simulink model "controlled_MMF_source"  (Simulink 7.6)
settings: Solver=ode15s  StartTime=0.0  StopTime=50  RelTol=1e-3
StopFcn:
  | load MMF_variable_pos_vit.mat
  | close all
  | plotyy(x(1,:),x(2,:),x(1,:),x(3,:))
  | grid
  | title('Position et vitesse de la masse')
  | 
  | figure
  | load MMF_variable_flux_MMF.mat
  | plotyy(y(1,:),y(2,:),y(1,:),y(3,:))
  | grid
  | title('Flux magnétique et MMF')
  | delete *.mat
undefined symbols (not defined in the file or in its folder): sigbuilder_block
libraries: fl_lib x12, nesl_utility x6

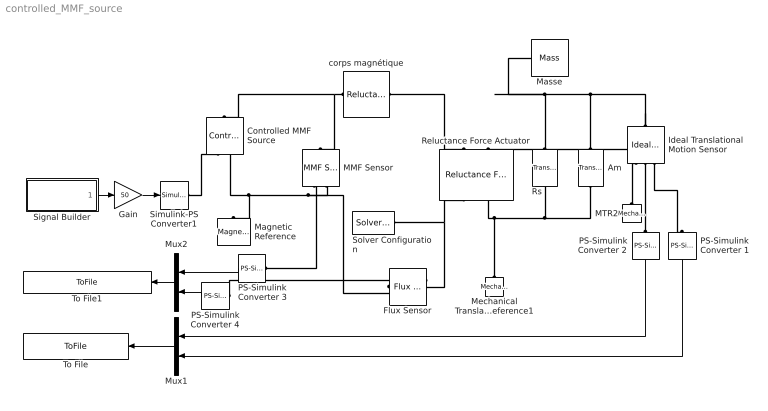
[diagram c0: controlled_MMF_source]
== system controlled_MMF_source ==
  Am : fl_lib/Mechanical/Translational Elements/Translational Damper  DialogController=NetworkEngine.DynNeDlgSource  SystemSampleTime=-1  D=10 N/(m/s)  f_Log=off  v_Log=off  LocalVarNames=|force|rel_velocity|power  LocalVarDescs=|Damping force (N)|Damper relative velocity (m/s)|Power dissipated in the damper (W)  LocalVarLogging=[0 0 0]
  Controlled MMF Source : fl_lib/Magnetic/Magnetic Sources/Controlled MMF Source  DialogController=NetworkEngine.DynNeDlgSource  SystemSampleTime=-1  phi_Log=off  mmf_Log=off  LocalVarNames=|phi|mmf  LocalVarDescs=|phi|mmf  LocalVarLogging=[0 0]
  Flux Sensor : fl_lib/Magnetic/Magnetic Sensors/Flux Sensor  DialogController=NetworkEngine.DynNeDlgSource  SystemSampleTime=-1  phi_Log=off  mmf_Log=off  LocalVarNames=|phi|mmf  LocalVarDescs=|phi|mmf  LocalVarLogging=[0 0]
  Gain : Gain  Gain=50
  Ideal Translational Motion Sensor : fl_lib/Mechanical/Mechanical Sensors/Ideal Translational Motion Sensor  DialogController=NetworkEngine.DynNeDlgSource  SystemSampleTime=-1  offset=5 mm  v_Log=off  f_Log=off  x_Log=off  LocalVarNames=|v|f|x  LocalVarDescs=|v|f|x  LocalVarLogging=[]
  MMF Sensor : fl_lib/Magnetic/Magnetic Sensors/MMF Sensor  DialogController=NetworkEngine.DynNeDlgSource  SystemSampleTime=-1  phi_Log=off  mmf_Log=off  LocalVarNames=|phi|mmf  LocalVarDescs=|phi|mmf  LocalVarLogging=[0 0]
  MTR2 : fl_lib/Mechanical/Translational Elements/Mechanical Translational Reference  Tag=Factory Generic  DialogController=NetworkEngine.DynNeDlgSource  SystemSampleTime=-1  f_Log=off  LocalVarNames=|f  LocalVarDescs=|f  LocalVarLogging=[]
  Magnetic Reference : fl_lib/Magnetic/Magnetic Elements/Magnetic Reference  DialogController=NetworkEngine.DynNeDlgSource  SystemSampleTime=-1  phi_Log=off  LocalVarNames=|phi  LocalVarDescs=|phi  LocalVarLogging=0
  Masse : fl_lib/Mechanical/Translational Elements/Mass  DialogController=NetworkEngine.DynNeDlgSource  SystemSampleTime=-1  mass=1 kg  initial_velocity=0 m/s  f_Log=off  LocalVarNames=|force|velocity  LocalVarDescs=|Inertia force (N)|Mass absolute velocity (m/s)  LocalVarLogging=[0 0]
  Mechanical Translational Reference1 : fl_lib/Mechanical/Translational Elements/Mechanical Translational Reference  DialogController=NetworkEngine.DynNeDlgSource  SystemSampleTime=-1  f_Log=off  LocalVarNames=|f  LocalVarDescs=|f  LocalVarLogging=[]
  Mux1 : Mux  Inputs=2
  Mux2 : Mux  Inputs=2
  PS-Simulink Converter 1 : nesl_utility/PS-Simulink Converter  DialogController=NetworkEngine.DynNeUtilDlgSource  SystemSampleTime=-1  PhysicalDomain=network_engine_domain  LeftPortType=input  RightPortType=output  SubClassName=ps_output  Unit=m  AffineConversion=off
  PS-Simulink Converter 2 : nesl_utility/PS-Simulink Converter  DialogController=NetworkEngine.DynNeUtilDlgSource  SystemSampleTime=-1  PhysicalDomain=network_engine_domain  LeftPortType=input  RightPortType=output  SubClassName=ps_output  Unit=m/s  AffineConversion=off
  PS-Simulink Converter 3 : nesl_utility/PS-Simulink Converter  DialogController=NetworkEngine.DynNeUtilDlgSource  SystemSampleTime=-1  PhysicalDomain=network_engine_domain  LeftPortType=input  RightPortType=output  SubClassName=ps_output  Unit=A  AffineConversion=off
  PS-Simulink Converter 4 : nesl_utility/PS-Simulink Converter  DialogController=NetworkEngine.DynNeUtilDlgSource  SystemSampleTime=-1  PhysicalDomain=network_engine_domain  LeftPortType=input  RightPortType=output  SubClassName=ps_output  Unit=Wb  AffineConversion=off
  Reluctance Force Actuator : fl_lib/Magnetic/Magnetic Elements/Reluctance Force Actuator  DialogController=NetworkEngine.DynNeDlgSource  SystemSampleTime=-1  x0=5 mm  xmin=1e-9 mm  CSA=4 cm^2  mur=1  K_contact=1e6 N/m  D_contact=50 N/(m/s)  mmf_Log=off  phi_Log=off  f_Log=off  u_Log=off  x_Log=off  LocalVarNames=|mmf|phi|f|u|x  LocalVarDescs=|mmf|phi|f|u|x  LocalVarLogging=[0 0 0 0 0]
  Rs : fl_lib/Mechanical/Translational Elements/Translational Spring  DialogController=NetworkEngine.DynNeDlgSource  SystemSampleTime=-1  spr_rate=150 N/m  init_def=0 mm  f_Log=off  v_Log=off  x_Log=off  LocalVarNames=|force|deformation  LocalVarDescs=|Spring force (N)|Spring deformation (m)  LocalVarLogging=[0 0]
  Signal Builder : Subsystem  Tag=STV Subsys  LoadFcn=sigbuilder_block('load');  StartFcn=sigbuilder_block('start');  StopFcn=sigbuilder_block('stop');  ClipboardFcn=sigbuilder_block('clipboard');
  Simulink-PS Converter1 : nesl_utility/Simulink-PS Converter  DialogController=NetworkEngine.DynNeUtilDlgSource  SystemSampleTime=-1  PhysicalDomain=network_engine_domain  LeftPortType=input  RightPortType=output  SubClassName=ps_input  Unit=1  AffineConversion=off  InputFilterTimeConstant=.001  UdotUserProvided=0
  Solver Configuration : nesl_utility/Solver Configuration  DialogController=NetworkEngine.DynNeUtilDlgSource  SystemSampleTime=-1  PhysicalDomain=network_engine_domain  LeftPortType=input  RightPortType=generic  SubClassName=solver  Accelerate=off  Profile=off  ResidualTolerance=1e-9  MaxNonlinIter=3  MaxModeIter=2  DoFixedCost=off  UseLocalSampling=off  DoDC=off  LinearAlgebra=Sparse  LocalSolverSampleTime=.001  LocalSolverChoice=NE_BACKWARD_EULER_ADVANCER  UseLocalSolver=off
  To File : ToFile  Filename=MMF_variable_pos_vit  MatrixName=x
  To File1 : ToFile  Filename=MMF_variable_flux_MMF  MatrixName=y
  corps magnétique : fl_lib/Magnetic/Magnetic Elements/Reluctance  DialogController=NetworkEngine.DynNeDlgSource  SystemSampleTime=-1  g=10 cm  CSA=10 cm^2  mur=50000  phi_Log=off  mmf_Log=off  LocalVarNames=|phi|mmf  LocalVarDescs=|phi|mmf  LocalVarLogging=[0 0]
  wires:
  Signal Builder/1(Signal 1) -> Gain/1
  PS-Simulink Converter 1/1 -> Mux1/2
  Mux1/1 -> To File/1
  Gain/1 -> Simulink-PS Converter1/1
  PS-Simulink Converter 2/1 -> Mux1/1
  PS-Simulink Converter 4/1 -> Mux2/2
  PS-Simulink Converter 3/1 -> Mux2/1
  Mux2/1 -> To File1/1
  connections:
  Ideal Translational Motion Sensor/LConn1 -- Am/LConn1 -- Rs/LConn1 -- Reluctance Force Actuator/LConn2 -- Masse/LConn1
  Am/RConn1 -- Reluctance Force Actuator/RConn2 -- Mechanical Translational Reference1/LConn1 -- Rs/RConn1
  corps magnétique/RConn1 -- Reluctance Force Actuator/LConn1
  PS-Simulink Converter 4/LConn1 -- Flux Sensor/RConn1
  Ideal Translational Motion Sensor/RConn3 -- PS-Simulink Converter 1/LConn1
  MTR2/LConn1 -- Ideal Translational Motion Sensor/RConn1
  corps magnétique/LConn1 -- Controlled MMF Source/LConn1 -- MMF Sensor/LConn1
  MMF Sensor/RConn2 -- Flux Sensor/RConn2 -- Controlled MMF Source/RConn2 -- Magnetic Reference/LConn1
  Simulink-PS Converter1/RConn1 -- Controlled MMF Source/RConn1
  PS-Simulink Converter 2/LConn1 -- Ideal Translational Motion Sensor/RConn2
  PS-Simulink Converter 3/LConn1 -- MMF Sensor/RConn1
  Solver Configuration/RConn1 -- Reluctance Force Actuator/RConn1 -- Flux Sensor/LConn1

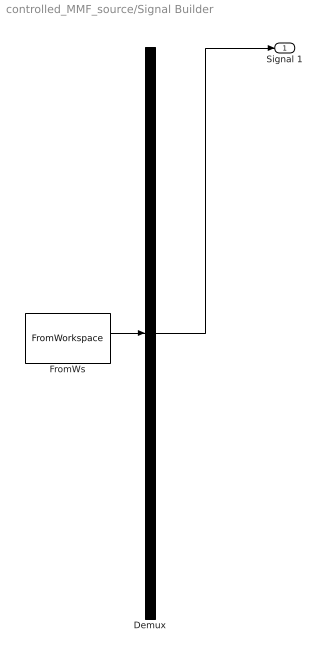
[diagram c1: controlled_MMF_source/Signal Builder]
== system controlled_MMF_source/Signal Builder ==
  Demux : Demux  Tag=STV Demux  Outputs=1
  FromWs : FromWorkspace  Tag=STV FromWs  VariableName=tuvar  SampleTime=0  SigBuilderData=DataTag0  VnvData=DataTag1
  Signal 1 : Outport  Tag=STV Outport
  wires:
  FromWs/1 -> Demux/1
  Demux/1 -> Signal 1/1
